(* Logix 5000 AddOnInstructionDefinition export SPEL_Oport; software revision 30.01 *)

ADD_ON_INSTRUCTION SPEL_ExecCmd   (* revision 1.0 *)
// Executes a command in the robot controller.  Normally this is called by higher level AOIs.
VAR_INPUT
   Start : BOOL; {required}
   MaxTime : DINT := 3000; {required}
END_VAR
VAR_OUTPUT
   InCycle : BOOL; {access Read Only, visible}
   Done : BOOL; {access Read Only, visible}
   Error : BOOL; {access Read Only, visible}
END_VAR
VAR_IN_OUT
   ExtInputs : AB:ETHERNET_MODULE_INT_128Bytes:I:0; {required}
        .DATA[0].0   // ExtCmdGet
        .DATA[0].1   // ExtRespSet
        .DATA[0].2   // ExtCmdResult
        .DATA[0].3   // ExtError
   ExtOutputs : AB:ETHERNET_MODULE_INT_128Bytes:O:0; {required}
        .DATA[0].0   // ExtCmdSet
        .DATA[0].1   // ExtRespGet
        .DATA[0].2   // ExtCmdReset
END_VAR
VAR_INPUT
   Cmd : INT; {required}
   CmdParam1 : INT; {required}
   CmdParam2 : INT; {required}
   CmdParam3 : INT; {required}
   CmdParam4 : INT; {required}
   CmdParam5 : INT; {required}
   CmdParam6 : INT; {required}
   CmdParam7 : INT; {required}
END_VAR
VAR_OUTPUT
   CmdEcho : INT; {access Read Only, visible}
   Resp1 : INT; {access Read Only, visible}
   Resp2 : INT; {access Read Only, visible}
   Resp3 : INT; {access Read Only, visible}
   Resp4 : INT; {access Read Only, visible}
   Resp5 : INT; {access Read Only, visible}
   Resp6 : INT; {access Read Only, visible}
   Resp7 : INT; {access Read Only, visible}
   ErrCode1 : INT; {access Read Only, visible}
   ErrCode2 : INT; {access Read Only, visible}
END_VAR
VAR
   ExtReset : BOOL; {access None}
   ExtError : BOOL; {access None}
   ExtCmdSet : BOOL; {access None}   // Cmd Ready
   ExtCmdGet : BOOL; {access None}   // Cmd Received
   CmdXferDone : BOOL; {access None}
   ExtRespSet : BOOL; {access None}   // Resp Ready
   RespXferDone : BOOL; {access None}
   ExtCmdResult : BOOL; {access None}   // Normal or Error?
   TmrCmdDataRdy : TIMER := (PRE := 5); {access None}
   OneShotDoneOff : BOOL; {access None}
   OneShotStart : BOOL; {access None}
   StartInit : BOOL; {access None}
   OneShotStartError : BOOL; {access None}
   TmrCycle : TIMER := (PRE := 5000); {access None}
   OneshotTmrPreset : BOOL; {access None}
   TmrCmdSet : TIMER := (PRE := 20); {access None}
   OnShotCmdDataXfer : BOOL; {access None}
   OneShotRespDataXfer : BOOL; {access None}
   OneShotDataRdy : BOOL; {access None}
   OtherCmdInCycle : BOOL; {access None}
   s : BOOL; {access None}
   OneShotUnsetCmdIncycle : BOOL; {access None}
   OneShotSetCmdIncycle : BOOL; {access None}
   OneShotSetOtherCmdInCycleError : BOOL; {access None}
   OneShotSetBit : BOOL; {access None}
END_VAR

ROUTINE Logic   (* ladder *)
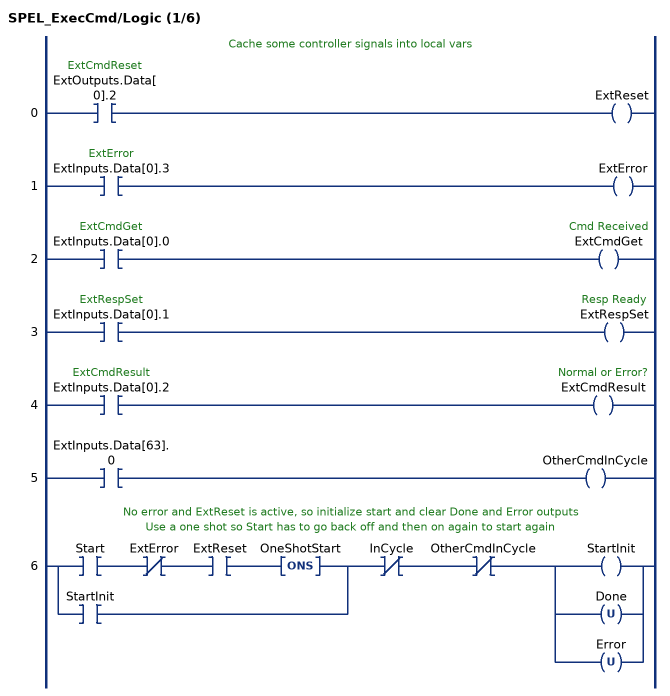
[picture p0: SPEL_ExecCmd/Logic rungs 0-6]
   // Cache some controller signals into local vars
   0: XIC(ExtOutputs.Data[0].2)OTE(ExtReset);
   1: XIC(ExtInputs.Data[0].3)OTE(ExtError);
   2: XIC(ExtInputs.Data[0].0)OTE(ExtCmdGet);
   3: XIC(ExtInputs.Data[0].1)OTE(ExtRespSet);
   4: XIC(ExtInputs.Data[0].2)OTE(ExtCmdResult);
   5: XIC(ExtInputs.Data[63].0)OTE(OtherCmdInCycle);
   // No error and ExtReset is active, so initialize start and clear Done and Error outputs
   // Use a one shot so Start has to go back off and then on again to start again
   6: [XIC(Start) XIO(ExtError) XIC(ExtReset) ONS(OneShotStart) ,XIC(StartInit) ]XIO(InCycle)XIO(OtherCmdInCycle)[OTE(StartInit) ,OTU(Done) ,OTU(Error) ];
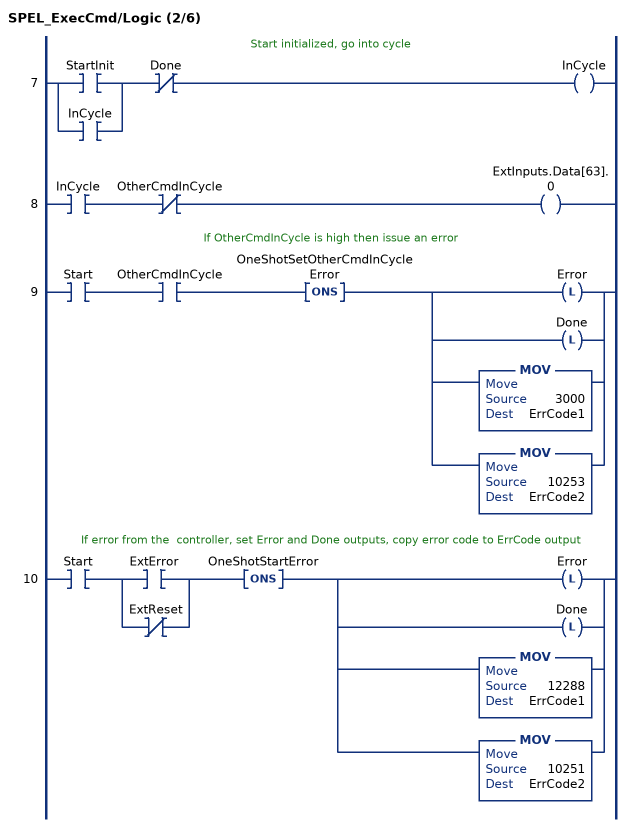
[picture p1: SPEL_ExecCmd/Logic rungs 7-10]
   // Start initialized, go into cycle
   7: [XIC(StartInit) ,XIC(InCycle) ]XIO(Done)OTE(InCycle);
   8: XIC(InCycle)XIO(OtherCmdInCycle)OTE(ExtInputs.Data[63].0);
   // If OtherCmdInCycle is high then issue an error
   9: XIC(Start)XIC(OtherCmdInCycle)ONS(OneShotSetOtherCmdInCycleError)[OTL(Error) ,OTL(Done) ,MOV(3000,ErrCode1) ,MOV(10253,ErrCode2) ];
   // If error from the  controller, set Error and Done outputs, copy error code to ErrCode output
   10: XIC(Start)[XIC(ExtError) ,XIO(ExtReset) ]ONS(OneShotStartError)[OTL(Error) ,OTL(Done) ,MOV(12288,ErrCode1) ,MOV(10251,ErrCode2) ];
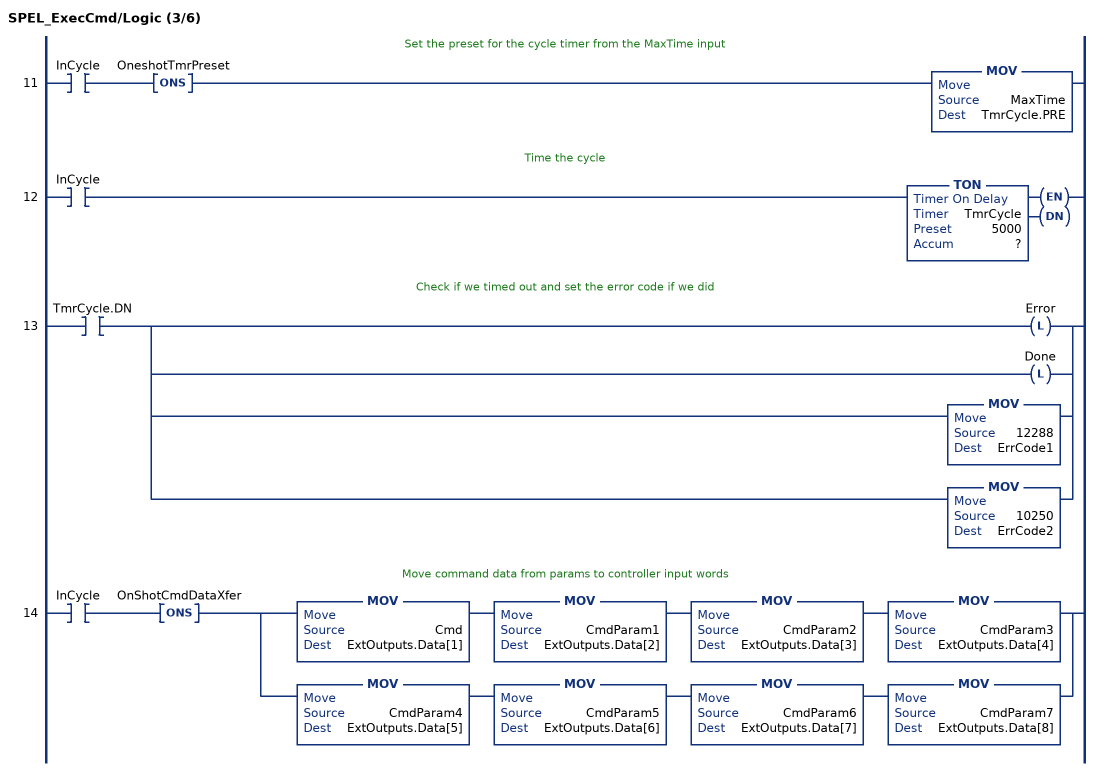
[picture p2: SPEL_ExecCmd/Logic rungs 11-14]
   // Set the preset for the cycle timer from the MaxTime input
   11: XIC(InCycle)ONS(OneshotTmrPreset)MOV(MaxTime,TmrCycle.PRE);
   // Time the cycle
   12: XIC(InCycle)TON(TmrCycle,?,?);
   // Check if we timed out and set the error code if we did
   13: XIC(TmrCycle.DN)[OTL(Error) ,OTL(Done) ,MOV(12288,ErrCode1) ,MOV(10250,ErrCode2) ];
   // Move command data from params to controller input words
   14: XIC(InCycle)ONS(OnShotCmdDataXfer)[MOV(Cmd,ExtOutputs.Data[1]) MOV(CmdParam1,ExtOutputs.Data[2]) MOV(CmdParam2,ExtOutputs.Data[3]) MOV(CmdParam3,ExtOutputs.Data[4]) ,MOV(CmdParam4,ExtOutputs.Data[5]) MOV(CmdParam5,ExtOutputs.Data[6]) MOV(CmdParam6,ExtOutputs.Data[7]) MOV(CmdParam7,ExtOutputs.Data[8]) ];
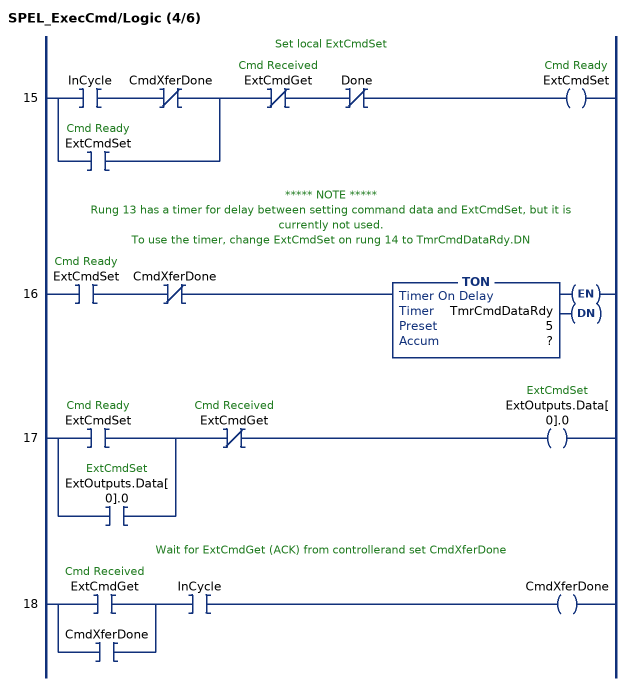
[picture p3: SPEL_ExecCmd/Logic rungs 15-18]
   // Set local ExtCmdSet
   15: [XIC(InCycle) XIO(CmdXferDone) ,XIC(ExtCmdSet) ]XIO(ExtCmdGet)XIO(Done)OTE(ExtCmdSet);
   // ***** NOTE *****
   // Rung 13 has a timer for delay between setting command data and ExtCmdSet, but it is currently not used.
   // To use the timer, change ExtCmdSet on rung 14 to TmrCmdDataRdy.DN
   16: XIC(ExtCmdSet)XIO(CmdXferDone)TON(TmrCmdDataRdy,?,?);
   17: [XIC(ExtCmdSet) ,XIC(ExtOutputs.Data[0].0) ]XIO(ExtCmdGet)OTE(ExtOutputs.Data[0].0);
   // Wait for ExtCmdGet (ACK) from controllerand set CmdXferDone
   18: [XIC(ExtCmdGet) ,XIC(CmdXferDone) ]XIC(InCycle)OTE(CmdXferDone);
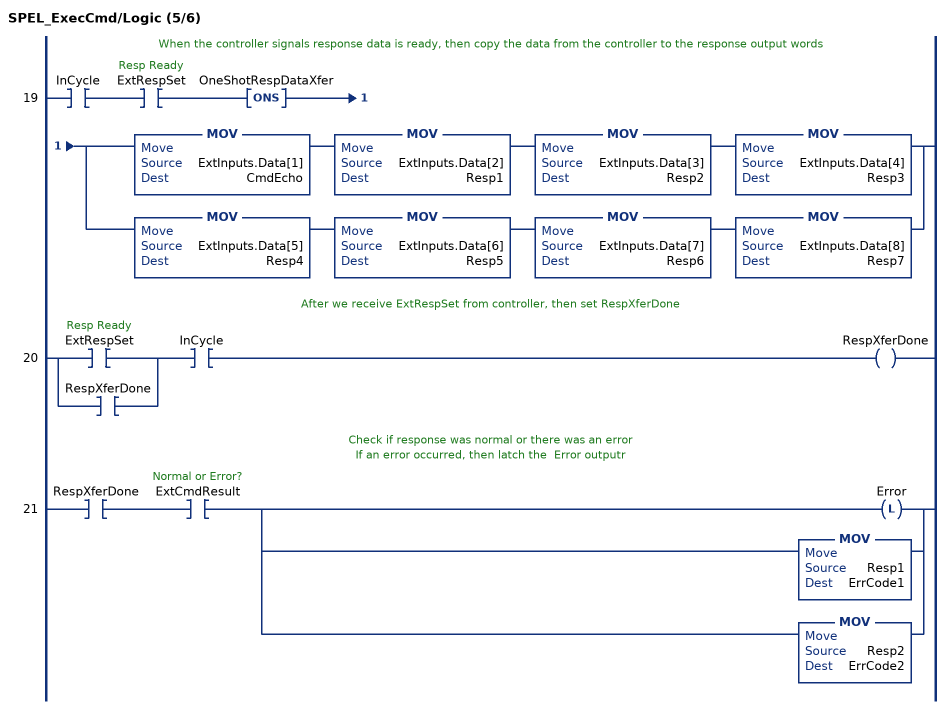
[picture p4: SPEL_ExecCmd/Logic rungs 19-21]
   // When the controller signals response data is ready, then copy the data from the controller to the response output words
   19: XIC(InCycle)XIC(ExtRespSet)ONS(OneShotRespDataXfer)[MOV(ExtInputs.Data[1],CmdEcho) MOV(ExtInputs.Data[2],Resp1) MOV(ExtInputs.Data[3],Resp2) MOV(ExtInputs.Data[4],Resp3) ,MOV(ExtInputs.Data[5],Resp4) MOV(ExtInputs.Data[6],Resp5) MOV(ExtInputs.Data[7],Resp6) MOV(ExtInputs.Data[8],Resp7) ];
   // After we receive ExtRespSet from controller, then set RespXferDone
   20: [XIC(ExtRespSet) ,XIC(RespXferDone) ]XIC(InCycle)OTE(RespXferDone);
   // Check if response was normal or there was an error
   // If an error occurred, then latch the  Error outputr
   21: XIC(RespXferDone)XIC(ExtCmdResult)[OTL(Error) ,MOV(Resp1,ErrCode1) ,MOV(Resp2,ErrCode2) ];
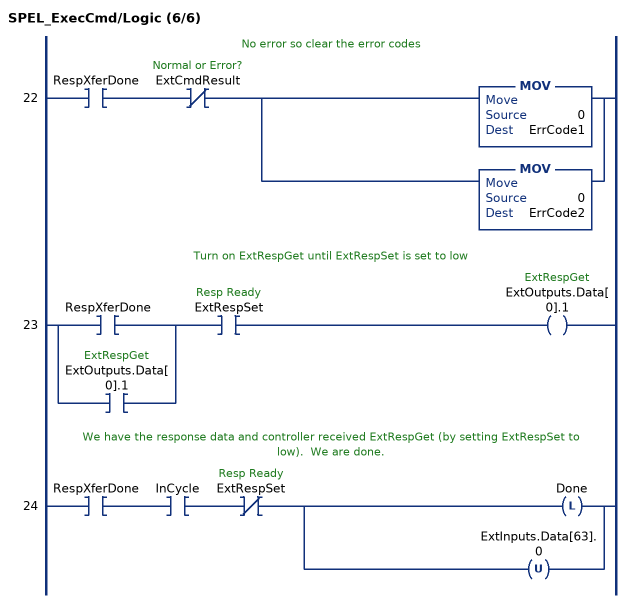
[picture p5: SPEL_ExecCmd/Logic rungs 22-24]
   // No error so clear the error codes
   22: XIC(RespXferDone)XIO(ExtCmdResult)[MOV(0,ErrCode1) ,MOV(0,ErrCode2) ];
   // Turn on ExtRespGet until ExtRespSet is set to low
   23: [XIC(RespXferDone) ,XIC(ExtOutputs.Data[0].1) ]XIC(ExtRespSet)OTE(ExtOutputs.Data[0].1);
   // We have the response data and controller received ExtRespGet (by setting ExtRespSet to low).  We are done.
   24: XIC(RespXferDone)XIC(InCycle)XIO(ExtRespSet)[OTL(Done) ,OTU(ExtInputs.Data[63].0) ];
END_ROUTINE
END_ADD_ON_INSTRUCTION

ADD_ON_INSTRUCTION SPEL_Oport   (* revision 1.2, vendor SEIKO EPSON CORP. *)
// Returns the state of the specified output bit.
VAR_INPUT
   Start : BOOL; {access None, required}
END_VAR
VAR_OUTPUT
   InCycle : BOOL; {access None, visible}
   Done : BOOL; {access Read Only, visible}
   Error : BOOL; {access None, visible}
END_VAR
VAR_INPUT
   BitNum : INT; {access None, required}
END_VAR
VAR_OUTPUT
   Status : INT; {access Read Only, visible}
END_VAR
VAR_IN_OUT
   ExtInputs : AB:ETHERNET_MODULE_INT_128Bytes:I:0; {required}
   ExtOutputs : AB:ETHERNET_MODULE_INT_128Bytes:O:0; {required}
END_VAR
VAR_OUTPUT
   ErrCode1 : INT; {access Read Only, visible}
   ErrCode2 : INT; {access Read Only, visible}
END_VAR
VAR
   ExecOport : SPEL_ExecCmd := (MaxTime := 3000); {access None}
END_VAR

ROUTINE Logic   (* ladder *)
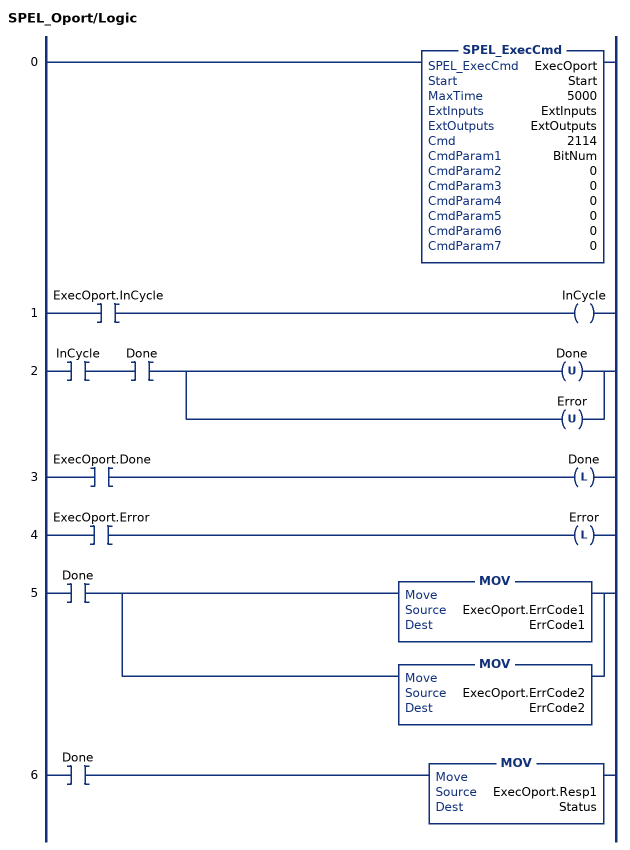
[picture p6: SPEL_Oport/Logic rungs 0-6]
   0: SPEL_ExecCmd(ExecOport,Start,5000,ExtInputs,ExtOutputs,2114,BitNum,0,0,0,0,0,0);
   1: XIC(ExecOport.InCycle)OTE(InCycle);
   2: XIC(InCycle)XIC(Done)[OTU(Done) ,OTU(Error) ];
   3: XIC(ExecOport.Done)OTL(Done);
   4: XIC(ExecOport.Error)OTL(Error);
   5: XIC(Done)[MOV(ExecOport.ErrCode1,ErrCode1) ,MOV(ExecOport.ErrCode2,ErrCode2) ];
   6: XIC(Done)MOV(ExecOport.Resp1,Status);
END_ROUTINE
END_ADD_ON_INSTRUCTION
